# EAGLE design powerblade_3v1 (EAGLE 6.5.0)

## Sheet 1 of 6: AC-DC Power Supply
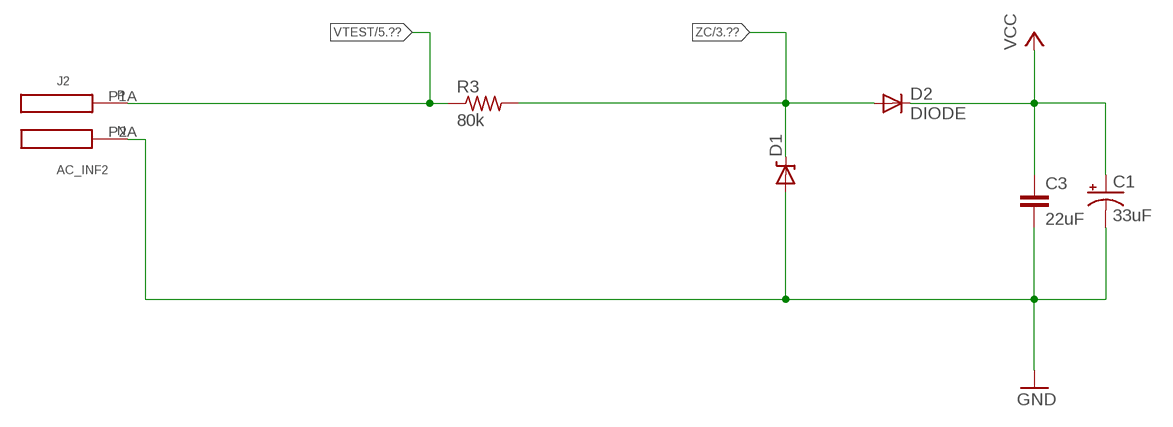
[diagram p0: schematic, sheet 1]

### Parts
C1  33uF  CPOL-US0805_SM  [CPOL0805_SM]
C3  22uF  C-EUC0603_SM  [C0603_SM]
D1  ZENERBZT52  [BZT52]
D2  DIODE  [BAS521]
J2  AC_INF2  [AC3_F2]
R3  80k  R-US_R1210  [R1210]

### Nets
GND: C1.- C3.2 D1.A J2.P2A(N) ; also sheet 2,3,4,5,6
VCC: C1.+ C3.1 D2.C ; also sheet 2,3,6
VTEST: J2.P1A(P) R3.1 ; also sheet 5
ZC: D1.C D2.A R3.2 ; also sheet 3,6

## Sheet 2 of 6: Load Supply Regulation
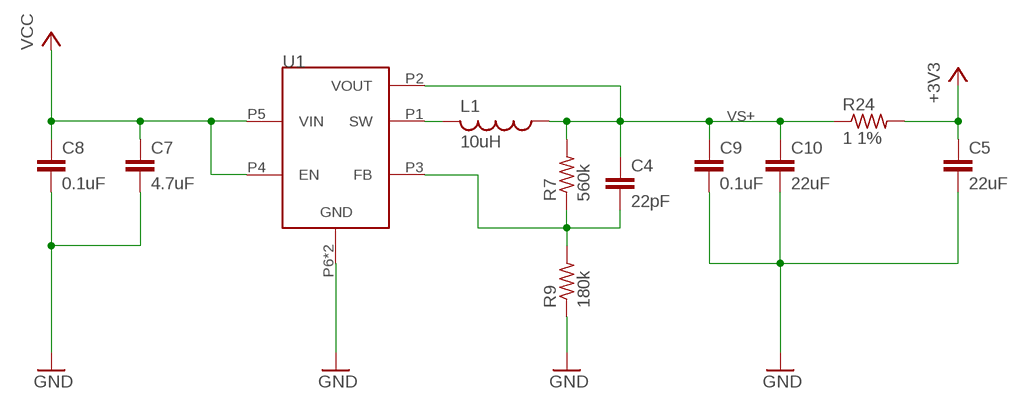
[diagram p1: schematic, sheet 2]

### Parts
C4  22pF  C-EUC0402_SM  [C0402_SM]
C5  22uF  C-EUC0603_TN  [C0603_TN]
C7  4.7uF  C-EUC0402_SM  [C0402_SM]
C8  0.1uF  C-EUC0402_SM  [C0402_SM]
C9  0.1uF  C-EUC0402_SM  [C0402_SM]
C10  22uF  C-EUC0603_SM  [C0603_SM]
L1  10uH  L-USL0805  [L0805]
R7  560k  R-US_R0402_SM  [R0402_SM]
R9  180k  R-US_R0402_SM  [R0402_SM]
R24  1 1%  R-US_R0603_SM  [R0603_SM]
U1  TPS62122  [WDFN-6]

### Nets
+3V3: C5.1 R24.2 ; also sheet 3,4,5,6
GND: C5.2 C7.2 C8.2 C9.2 C10.2 R9.1 U1.P6(GND) U1.PAD(GND) ; also sheet 1,3,4,5,6
N$9: L1.2 U1.P1(SW)
N$13: C4.2 R7.1 R9.2 U1.P3(FB)
VCC: C7.1 C8.1 U1.P4(EN) U1.P5(VIN) ; also sheet 1,3,6
VS+: C4.1 C9.1 C10.1 L1.1 R7.2 R24.1 U1.P2(VOUT) ; also sheet 6

## Sheet 3 of 6: MSP430FR5738
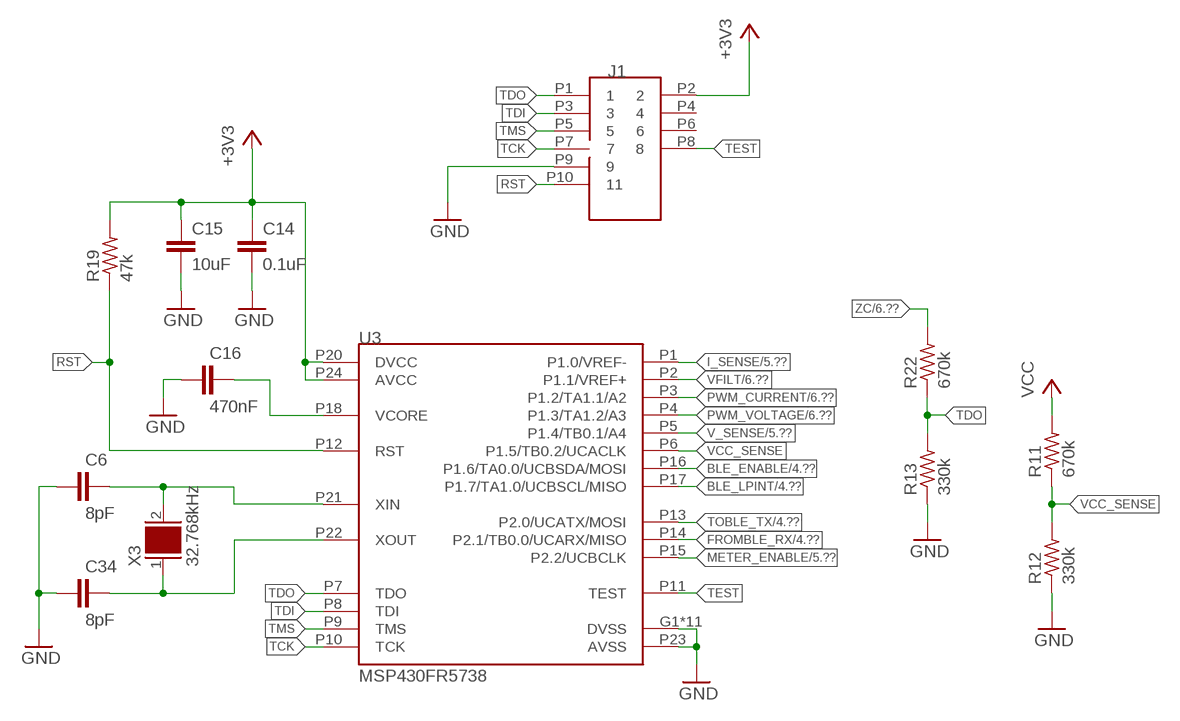
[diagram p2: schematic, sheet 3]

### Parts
C6  8pF  C-EUC0402_SM  [C0402_SM]
C14  0.1uF  C-EUC0402_SM  [C0402_SM]
C15  10uF  C-EUC0603_SM  [C0603_SM]
C16  470nF  C-EUC0402_SM  [C0402_SM]
C34  8pF  C-EUC0402_SM  [C0402_SM]
J1  JTAG_14PIN_IDC-ND  [TC2050-IDC-NL-430-ND]
R11  670k  R-US_R0402_SM  [R0402_SM]
R12  330k  R-US_R0402_SM  [R0402_SM]
R13  330k  R-US_R0402_SM  [R0402_SM]
R19  47k  R-US_R0402_SM  [R0402_SM]
R22  670k  R-US_R0402_SM  [R0402_SM]
U3  MSP430FR5738  [VQFN-24]
X3  32.768kHz  CRYSTAL_0805  [0805]

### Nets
+3V3: C14.1 C15.1 J1.P2 R19.2 U3.P20(DVCC) U3.P24(AVCC) ; also sheet 2,4,5,6
BLE_ENABLE: U3.P16(P1.6/TA0.0/UCBSDA/MOSI) ; also sheet 4
BLE_LPINT: U3.P17(P1.7/TA1.0/UCBSCL/MISO) ; also sheet 4
FROMBLE_RX: U3.P14(P2.1/TB0.0/UCARX/MISO) ; also sheet 4,6
GND: C6.1 C14.2 C15.2 C16.1 C34.1 J1.P9 R12.1 R13.1 U3.G1(DVSS) U3.G2(DVSS) U3.G3(DVSS) U3.G4(DVSS) U3.G5(DVSS) U3.G6(DVSS) U3.G7(DVSS) U3.G8(DVSS) U3.G9(DVSS) U3.P19(DVSS) U3.P23(AVSS) U3.PAD(DVSS) ; also sheet 1,2,4,5,6
I_SENSE: U3.P1(P1.0/VREF-) ; also sheet 5,6
METER_ENABLE: U3.P15(P2.2/UCBCLK) ; also sheet 5
N$3: C34.2 U3.P22(XOUT) X3.1
N$23: C16.2 U3.P18(VCORE)
N$56: C6.2 U3.P21(XIN) X3.2
PWM_CURRENT: U3.P3(P1.2/TA1.1/A2) ; also sheet 6
PWM_VOLTAGE: U3.P4(P1.3/TA1.2/A3) ; also sheet 6
RST: J1.P10 R19.1 U3.P12(RST)
TCK: J1.P7 U3.P10(TCK)
TDI: J1.P3 U3.P8(TDI)
TDO: J1.P1 R13.2 R22.1 U3.P7(TDO)
TEST: J1.P8 U3.P11(TEST)
TMS: J1.P5 U3.P9(TMS)
TOBLE_TX: U3.P13(P2.0/UCATX/MOSI) ; also sheet 4,6
V_SENSE: U3.P5(P1.4/TB0.1/A4) ; also sheet 5,6
VCC: R11.2 ; also sheet 1,2,6
VCC_SENSE: R11.1 R12.2 U3.P6(P1.5/TB0.2/UCACLK)
VFILT: U3.P2(P1.1/VREF+) ; also sheet 5,6
ZC: R22.2 ; also sheet 1,6
Unconnected: J1.P4 J1.P6

## Sheet 4 of 6: nr51822
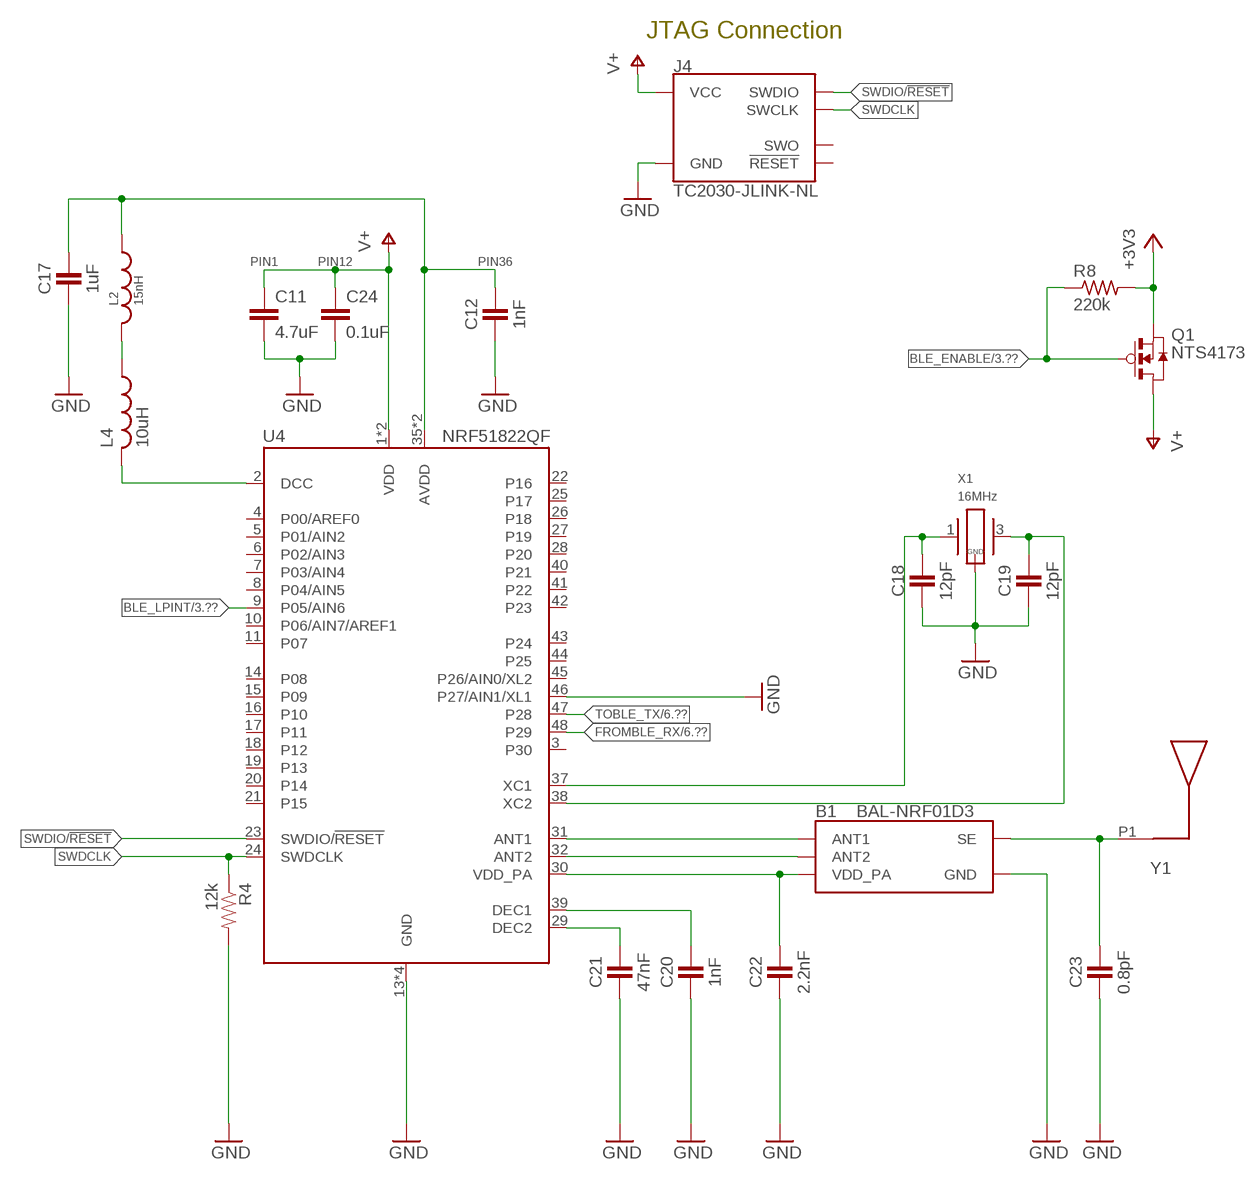
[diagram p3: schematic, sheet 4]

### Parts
B1  BAL-NRF01D3  [BAL-NRF01D3]
C11  4.7uF  C-EUC0402_SM  [C0402_SM]
C12  1nF  CAPACITOR  [0402_CAP]
C17  1uF  CAPACITOR  [0402_CAP]
C18  12pF  CAPACITOR  [0402_CAP]
C19  12pF  CAPACITOR  [0402_CAP]
C20  1nF  CAPACITOR  [0402_CAP]
C21  47nF  CAPACITOR  [0402_CAP]
C22  2.2nF  CAPACITOR  [0402_CAP]
C23  0.8pF  CAPACITOR  [0402_CAP]
C24  0.1uF  C-EUC0402_SM  [C0402_SM]
J4  TC2030-JLINK-NL  [TC2030-IDC-NL]
L2  15nH  INDUCTOR0402  [0402_CAP]
L4  10uH  L-USL0603_TN  [C0603_TN]
Q1  NTS4173  [SC-70-3]
R4  12k  RESISTOR  [0402_RES]
R8  220k  R-US_R0402_SM  [R0402_SM]
U4  NRF51822QF  [QFN-48-6MM]
X1  16MHz  TXC-8Y  [TXC-8Y]
Y1  UREACH_XTEND  [UREACH_XTEND]

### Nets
+3V3: Q1.P2(S) R8.2 ; also sheet 2,3,5,6
AVDD: C12.1 C17.1 L2.1 U4.35(AVDD) U4.36(AVDD)
BLE_ENABLE: Q1.P1(G) R8.1 ; also sheet 3
BLE_LPINT: U4.9(P05/AIN6) ; also sheet 3
DCC: L4.2 U4.2(DCC)
FROMBLE_RX: U4.48(P29) ; also sheet 3,6
GND: B1.GND C11.2 C12.2 C17.2 C18.2 C19.2 C20.2 C21.2 C22.2 C23.2 C24.2 J4.5(GND) R4.2 U4.13(GND) U4.33(GND) U4.34(GND) U4.46(P27/AIN1/XL1) U4.GND X1.2(GND) X1.4(GND) ; also sheet 1,2,3,5,6
N$4: B1.SE C23.1 Y1.P1
N$5: B1.ANT1 U4.31(ANT1)
N$6: B1.ANT2 U4.32(ANT2)
N$10: L2.2 L4.1
N$16: C18.1 U4.37(XC1) X1.1
N$17: C19.1 U4.38(XC2) X1.3
N$18: C20.1 U4.39(DEC1)
N$19: C21.1 U4.29(DEC2)
SWDCLK: J4.4(SWCLK) R4.1 U4.24(SWDCLK)
SWDIO/!RESET: J4.2(SWDIO) U4.23(SWDIO/!RESET)
TOBLE_TX: U4.47(P28) ; also sheet 3,6
V+: C11.1 C24.1 J4.1(VCC) Q1.P3(D) U4.1(VDD) U4.12(VDD)
VDD_PA: B1.VCC(VDD_PA) C22.1 U4.30(VDD_PA)
Unconnected: J4.3(!RESET) J4.6(SWO) U4.3(P30) U4.4(P00/AREF0) U4.5(P01/AIN2) U4.6(P02/AIN3) U4.7(P03/AIN4) U4.8(P04/AIN5) U4.10(P06/AIN7/AREF1) U4.11(P07) U4.14(P08) U4.15(P09) U4.16(P10) U4.17(P11) U4.18(P12) U4.19(P13) U4.20(P14) U4.21(P15) U4.22(P16) U4.25(P17) U4.26(P18) U4.27(P19) U4.28(P20) U4.40(P21) U4.41(P22) U4.42(P23) U4.43(P24) U4.44(P25) U4.45(P26/AIN0/XL2)

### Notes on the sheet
- JTAG Connection
- PIN1 | PIN12 | PIN36

## Sheet 5 of 6: Power Sensing!
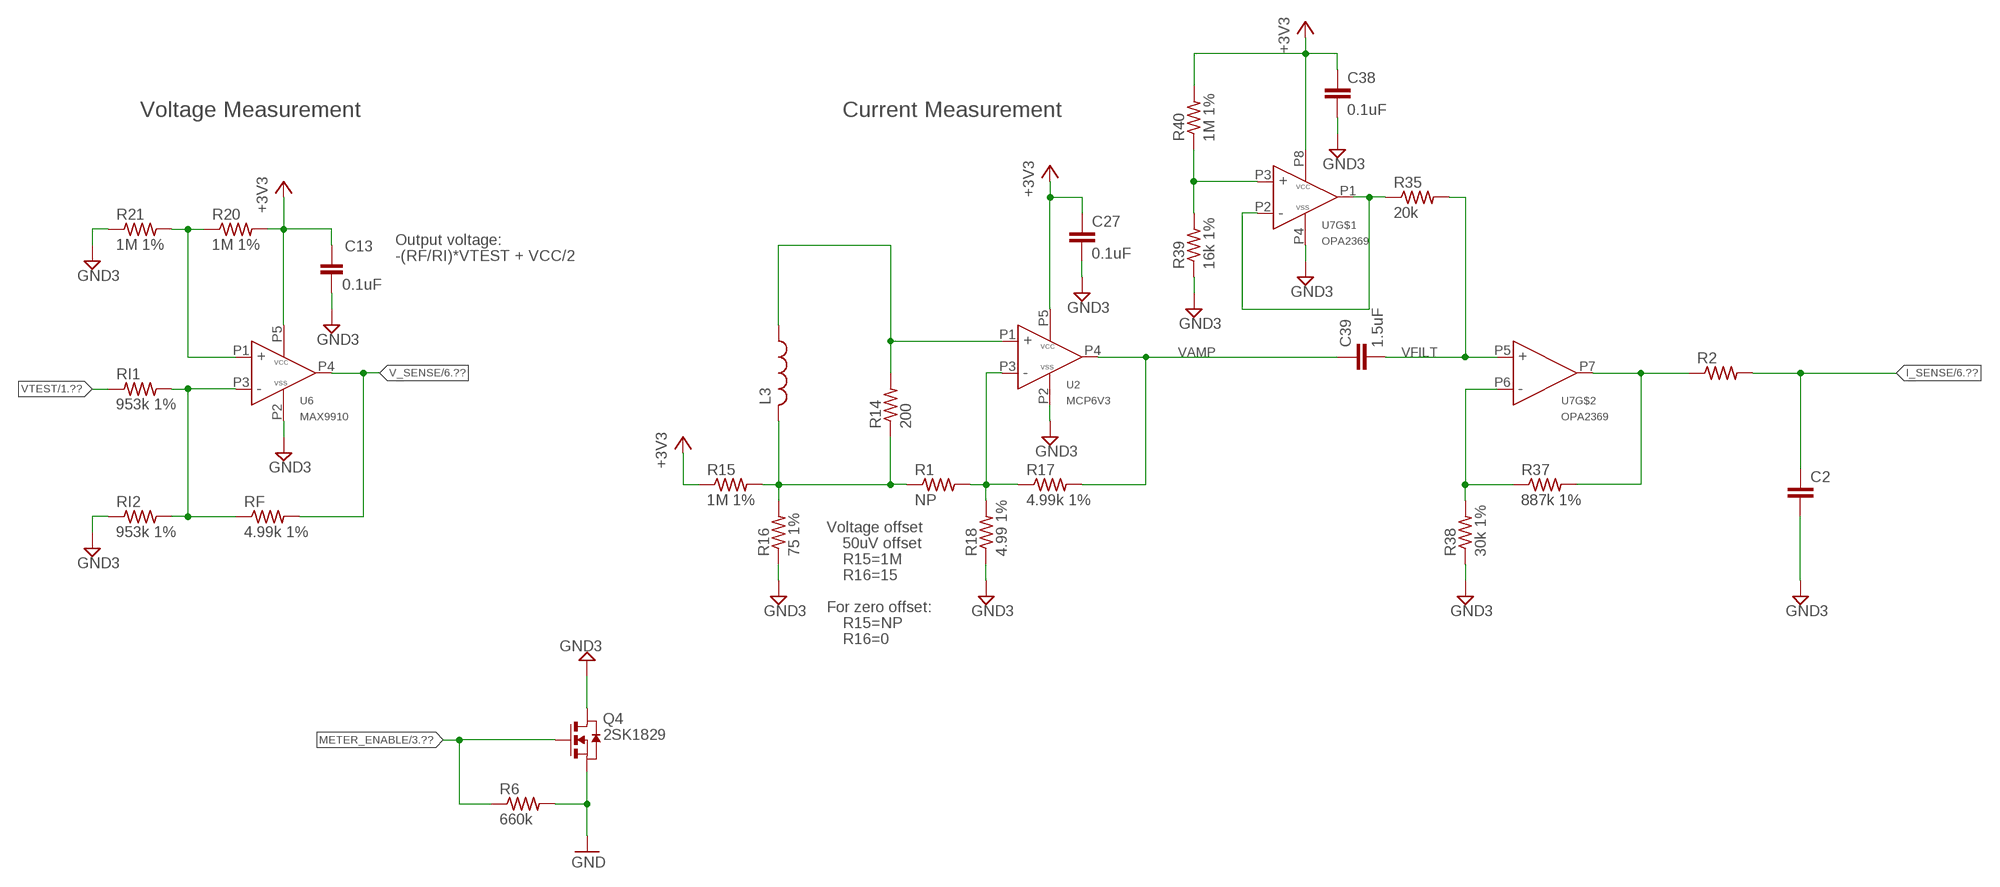
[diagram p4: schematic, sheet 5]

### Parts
C2  C-EUC0402_SM  [C0402_SM]
C13  0.1uF  CAPACITOR  [0402_CAP]
C27  0.1uF  C-EUC0402_SM  [C0402_SM]
C38  0.1uF  C-EUC0402_SM  [C0402_SM]
C39  1.5uF  C-EUC0402_SM  [C0402_SM]
L3  L-USL0805  [L0805]
Q4  2SK1829  [SC-70-3]
R1  NP  R-US_R0402_SM  [R0402_SM]
R2  R-US_R0402_SM  [R0402_SM]
R6  660k  R-US_R0402_SM  [R0402_SM]
R14  200  R-US_R0402_SM  [R0402_SM]
R15  1M 1%  R-US_R0402_SM  [R0402_SM]
R16  75 1%  R-US_R0402_SM  [R0402_SM]
R17  4.99k 1%  R-US_R0402_SM  [R0402_SM]
R18  4.99 1%  R-US_R0402_SM  [R0402_SM]
R20  1M 1%  R-US_R0402_SM  [R0402_SM]
R21  1M 1%  R-US_R0402_SM  [R0402_SM]
R35  20k  R-US_R0402_SM  [R0402_SM]
R37  887k 1%  R-US_R0402_SM  [R0402_SM]
R38  30k 1%  R-US_R0402_SM  [R0402_SM]
R39  16k 1%  R-US_R0402_SM  [R0402_SM]
R40  1M 1%  R-US_R0402_SM  [R0402_SM]
RF  4.99k 1%  R-US_R0402_SM  [R0402_SM]
RI1  953k 1%  R-US_R0402_SM  [R0402_SM]
RI2  953k 1%  R-US_R0402_SM  [R0402_SM]
U2  MCP6V3  [SC70-5]
U6  MAX9910  [SC70-5]
U7  OPA2369  [SOT-23-8]

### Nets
+3V3: C13.1 C27.1 C38.1 R15.1 R20.2 R40.2 U2.P5(VCC) U6.P5(VCC) U7.P8(VCC) ; also sheet 2,3,4,6
GND: Q4.P2(S) R6.2 ; also sheet 1,2,3,4,6
GND3: C2.2 C13.2 C27.2 C38.2 Q4.P3(D) R16.1 R18.1 R21.1 R38.1 R39.1 RI2.1 U2.P2(VSS) U6.P2(VSS) U7.P4(VSS)
I_SENSE: C2.1 R2.2 ; also sheet 3,6
METER_ENABLE: Q4.P1(G) R6.1 ; also sheet 3
N$1: R2.1 R37.2 U7.P7(OUT)
N$37: L3.2 R1.1 R14.1 R15.2 R16.2
N$38: L3.1 R14.2 U2.P1(IN+)
N$40: R20.1 R21.2 U6.P1(IN+)
N$41: RF.1 RI1.2 RI2.2 U6.P3(IN-)
N$65: R1.2 R17.1 R18.2 U2.P3(IN-)
N$66: R37.1 R38.2 U7.P6(IN-)
N$68: R35.1 U7.P1(OUT) U7.P2(IN-)
N$70: R39.2 R40.1 U7.P3(IN+)
V_SENSE: RF.2 U6.P4(OUT) ; also sheet 3,6
VAMP: C39.1 R17.2 U2.P4(OUT)
VFILT: C39.2 R35.2 U7.P5(IN+) ; also sheet 3,6
VTEST: RI1.1 ; also sheet 1

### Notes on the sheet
- Voltage Measurement | Current Measurement
- Output voltage:
- -(RF/RI)*VTEST + VCC/2
- Voltage offset
- 50uV offset
- R15=1M
- R16=15
- For zero offset:
- R15=NP
- R16=0

## Sheet 6 of 6: Debugging Connector. OOF
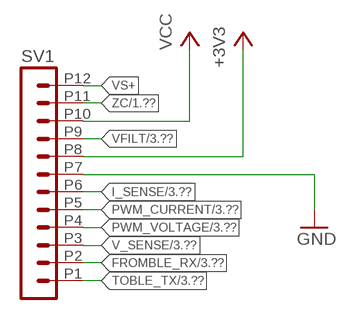
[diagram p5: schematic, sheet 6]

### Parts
SV1  MA12-11M27  [MA12-1_1MM27]

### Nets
+3V3: SV1.P8 ; also sheet 2,3,4,5
FROMBLE_RX: SV1.P2 ; also sheet 3,4
GND: SV1.P7 ; also sheet 1,2,3,4,5
I_SENSE: SV1.P6 ; also sheet 3,5
PWM_CURRENT: SV1.P5 ; also sheet 3
PWM_VOLTAGE: SV1.P4 ; also sheet 3
TOBLE_TX: SV1.P1 ; also sheet 3,4
V_SENSE: SV1.P3 ; also sheet 3,5
VCC: SV1.P10 ; also sheet 1,2,3
VFILT: SV1.P9 ; also sheet 3,5
VS+: SV1.P12 ; also sheet 2
ZC: SV1.P11 ; also sheet 1,3

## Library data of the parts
B1 = chips:BAL-NRF01D3: 50 ohm nominal input / conjugate match balun to nRF51422-QFAA, nRF24LE1, nRF51822-QFAA/AB, with integrated harmonic filter; DIGIKEY: 497-13637-1-ND; MOUSER: 511-BAL-NRF01D3
C1 = rcl:CPOL-US: POLARIZED CAPACITOR, American symbol; DIGIKEY: 478-8650-1-ND; DIGIKEY_2: 478-8654-1-ND
C2 = rcl:C-EU: CAPACITOR, European symbol
C3 C5 C10 = rcl:C-EU: CAPACITOR, European symbol; DIGIKEY: 445-9077-1-ND
C4 = rcl:C-EU: CAPACITOR, European symbol; DIGIKEY: 445-1239-1-ND
C6 C34 = rcl:C-EU: CAPACITOR, European symbol; DIGIKEY: 445-4890-1-ND
C7 = rcl:C-EU: CAPACITOR, European symbol; DIGIKEY: 445-8023-1-ND
C8 C9 C14 C24 C27 C38 = rcl:C-EU: CAPACITOR, European symbol; DIGIKEY: 445-4952-1-ND
C11 = rcl:C-EU: CAPACITOR, European symbol; DIGIKEY: 445-5947-1-ND
C12 C20 = passives:CAPACITOR: 0402 Capacitor; DIGIKEY: 490-1303-1-ND
C13 = passives:CAPACITOR: 0402 Capacitor; DIGIKEY: 445-4952-1-ND
C15 = rcl:C-EU: CAPACITOR, European symbol; DIGIKEY: 445-6853-1-ND
C16 = rcl:C-EU: CAPACITOR, European symbol; DIGIKEY: 445-4989-1-ND
C17 = passives:CAPACITOR: 0402 Capacitor; DIGIKEY: 1276-1513-1-ND
C18 C19 = passives:CAPACITOR: 0402 Capacitor; DIGIKEY: 490-6197-1-ND
C21 = passives:CAPACITOR: 0402 Capacitor; DIGIKEY: 445-1264-1-ND
C22 = passives:CAPACITOR: 0402 Capacitor; DIGIKEY: 490-5419-1-ND
C23 = passives:CAPACITOR: 0402 Capacitor; DIGIKEY: 490-6269-1-ND
C39 = rcl:C-EU: CAPACITOR, European symbol; DIGIKEY: 445-13815-1-ND
D1 = powerfilm:ZENER; DIGIKEY: BZT52C10T-7DICT-ND
D2 = powerfilm:DIODE; DIGIKEY: BAS521-7DICT-ND
J1 = ibat:JTAG_14PIN; DIGIKEY: NP
J2 = powerfilm:AC_IN; DIGIKEY: NP
J4 = connector:TC2030-JLINK; DIGIKEY: NP
L1 = rcl:L-US: INDUCTOR, American symbol; DIGIKEY: 490-4990-1-ND
L2 = passives:INDUCTOR; DIGIKEY: 587-1521-1-ND
L3 = rcl:L-US: INDUCTOR, American symbol; DIGIKEY: 732-3452-1-ND
L4 = rcl:L-US: INDUCTOR, American symbol; DIGIKEY: 490-4025-1-ND
Q1 = powerfilm:NTS4173; DIGIKEY: NTS4173PT1GOSCT-ND
Q4 = powerfilm:2SK1829; DIGIKEY: 2SK1829TE85LFCT-ND
R1 = rcl:R-US_: RESISTOR, American symbol; DIGIKEY: NP; DIGIKEY_2: P0.0JCT-ND
R2 = rcl:R-US_: RESISTOR, American symbol
R3 = rcl:R-US_: RESISTOR, American symbol; DIGIKEY: P80.6KAACT-ND; DIGIKEY_2: P69.8KAACT-ND; DIGIKEY_3: P40.2KAACT-ND
R4 = passives:RESISTOR: Resistor; DIGIKEY: RHM12.0KCDCT-ND
R6 R11 R22 = rcl:R-US_: RESISTOR, American symbol; DIGIKEY: P665KLCT-ND
R7 = rcl:R-US_: RESISTOR, American symbol; DIGIKEY: P560KLCT-ND
R8 = rcl:R-US_: RESISTOR, American symbol; DIGIKEY: P220KJCT-ND
R9 = rcl:R-US_: RESISTOR, American symbol; DIGIKEY: P180KLCT-ND
R12 R13 = rcl:R-US_: RESISTOR, American symbol; DIGIKEY: P330KLCT-ND
R14 = rcl:R-US_: RESISTOR, American symbol; DIGIKEY: P200LCT-ND
R15 R20 R21 R40 = rcl:R-US_: RESISTOR, American symbol; DIGIKEY: P1.00MLCT-ND
R16 = rcl:R-US_: RESISTOR, American symbol; DIGIKEY: P75.0LCT-ND
R17 = rcl:R-US_: RESISTOR, American symbol; DIGIKEY: P4.99KLCT-ND; DIGIKEY_2: P10.0KLCT-ND
R18 = rcl:R-US_: RESISTOR, American symbol; DIGIKEY: RMCF0402FT4R99CT-ND; DIGIKEY_2: P10.0LCT-ND
R19 = rcl:R-US_: RESISTOR, American symbol; DIGIKEY: P47KJCT-ND
R24 = rcl:R-US_: RESISTOR, American symbol; DIGIKEY: P1.0AJCT-ND
R35 = rcl:R-US_: RESISTOR, American symbol; DIGIKEY: P2.00KLCT-ND; DIGIKEY_2: P20.0KLCT-ND
R37 = rcl:R-US_: RESISTOR, American symbol; DIGIKEY: P887KLCT-ND
R38 = rcl:R-US_: RESISTOR, American symbol; DIGIKEY: P30.0KLCT-ND
R39 = rcl:R-US_: RESISTOR, American symbol; DIGIKEY: P16.0KLCT-ND
RF = rcl:R-US_: RESISTOR, American symbol; DIGIKEY: P4.99KLCT-ND
RI1 RI2 = rcl:R-US_: RESISTOR, American symbol; DIGIKEY: P953KLCT-ND
SV1 = con-lstb:MA12-1: PIN HEADER; DIGIKEY: S9014E-12-ND
U1 = powerfilm:TPS62122; DIGIKEY: 296-27695-1-ND
U2 = powerfilm:MCP6V3; DIGIKEY: MCP6V31UT-E/LTCT-ND; DIGIKEY_POP: 296-19547-1-ND
U3 = powerfilm:MSP430FR5738; DIGIKEY: 296-29232-1-ND
U4 = chips:NRF51822: Multiprotocol Bluetooth® 4.0 low energy/2.4 GHz RF SoC; DIGIKEY: 1490-1032-1-ND; MOUSER: 949-NRF51822-QFAB-R7
U6 = powerfilm:MAX9910; DIGIKEY: 296-25252-1-ND
U7 = powerfilm:OPA2369; DIGIKEY: 296-22671-1-ND
X1 = crystals:TXC-8Y: 2mmx1.6mm SMD Crystal; DIGIKEY: 887-2003-1-ND
X3 = general:CRYSTAL_0805; DIGIKEY: 535-12373-1-ND
Y1 = powerfilm:UREACH_XTEND; FRACTUS: FR05-S1-N-0-110

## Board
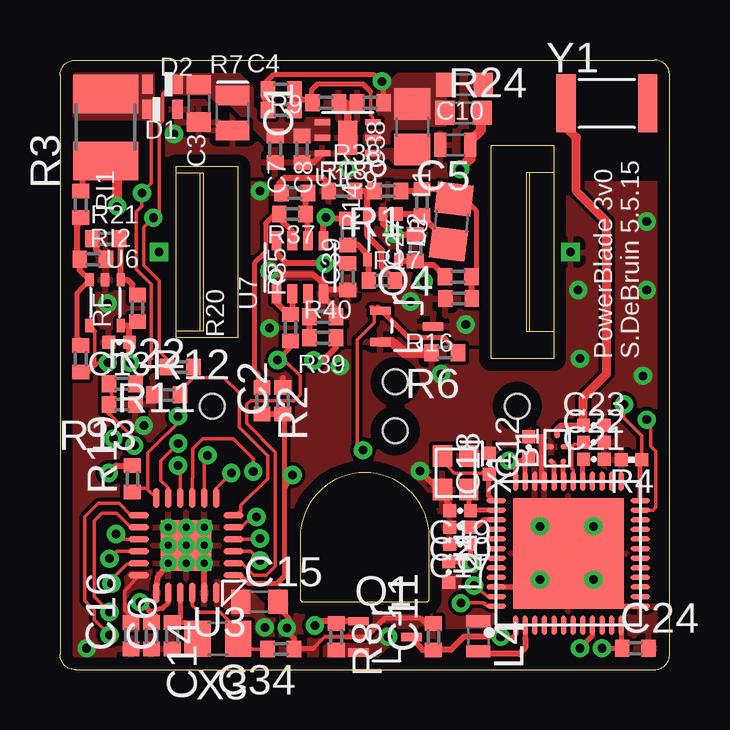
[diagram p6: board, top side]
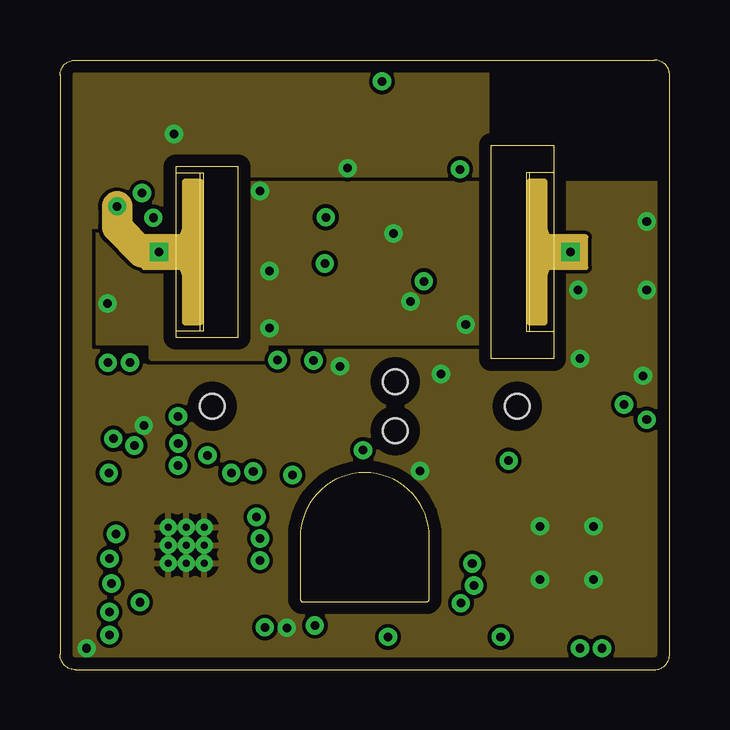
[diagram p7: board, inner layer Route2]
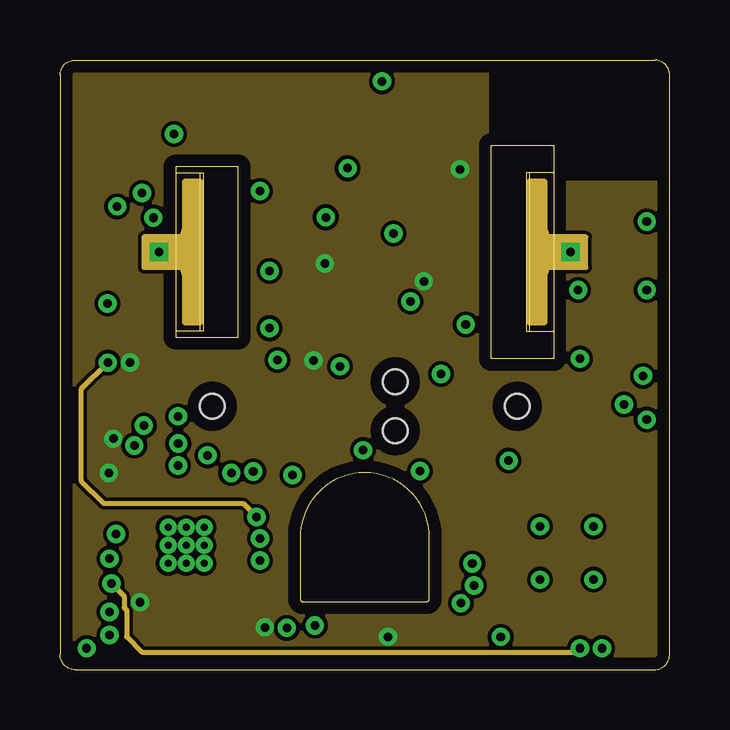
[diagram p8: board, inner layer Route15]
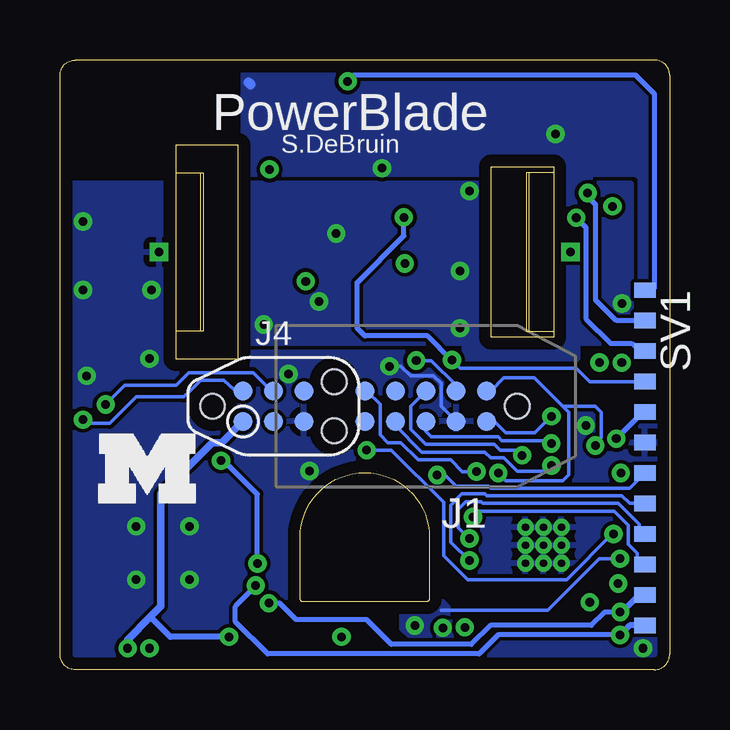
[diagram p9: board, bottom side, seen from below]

Size 25.4 x 25.4 mm. Coordinates in mm from the lower left corner, seen from the top.
Copper layers (1+2*15+16): Top 0.0178mm / dielectric 12mil / Route2 0.0356mm / dielectric 28mil / Route15 0.0356mm / dielectric 12mil / Bottom 0.0178mm
Design rules "SSC-EAGLE-4Lyr_v1.0.0.3 *": minimum track width 6mil, minimum drill 8mil, track to track 6mil, track to pad 6mil, pad to pad 6mil, via to via 6mil, smd to smd 6mil, copper to edge 20mil, drill to drill 16mil, minimum pad ring 8mil, minimum via ring 8mil, stop-mask expansion 3mil, vias tented up to drill 0mil, thermal gap 10mil

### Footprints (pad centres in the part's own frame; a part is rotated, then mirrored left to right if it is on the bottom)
BAL-NRF01D3 = smd 0.22 x 0.22: ANT1 -0.537,-0.25; ANT2 -0.537,0.25; GND 0.069,0.25; SE 0.537,0; VCC 0.069,-0.25
CPOL0805_SM = smd 0.8 x 1.4: + -0.73,0; - 0.73,0
C0402_SM = smd 0.6 x 0.7: 1 -0.55,0; 2 0.55,0
C0603_SM = smd 0.8 x 1: 1 -0.775,0; 2 0.775,0
C0603_TN = smd 0.5 x 1: 1 -0.625,0; 2 0.625,0
0402_CAP = smd 0.536 x 0.546: 1 -0.433,0; 2 0.433,0
BZT52 = smd 0.45 x 0.8: A -0.625,0; C 0.625,0
BAS521 = smd 0.45 x 0.8: A -0.625,0; C 0.625,0
TC2050-IDC-NL-430-ND = smd 0.787 x 0.787: P1 -2.54,-0.635; P2 -1.27,-0.635; P3 0,-0.635; P4 1.27,-0.635; P5 2.54,-0.635; P6 2.54,0.635; P7 1.27,0.635; P8 0,0.635; P9 -1.27,0.635; P10 -2.54,0.635 | hole 1.029: -3.81,0
AC3_F2 = drill 0.356 square: P1A -8.572,0; P2A 8.572,0
TC2030-IDC-NL = smd 0.787 x 0.787: 1 -1.27,-0.635; 2 -1.27,0.635; 3 0,-0.635; 4 0,0.635; 5 1.27,-0.635; 6 1.27,0.635 | hole 1.016: -2.54,0; 2.54,1.016; 2.54,-1.016
L0805 = smd 1.3 x 1.5: 1 -0.95,0; 2 0.95,0
SC-70-3 = smd 0.85 x 0.35: P1 -1.1,0.65; P2 -1.1,-0.65; P3 1.1,0
R0402_SM = smd 0.6 x 0.7: 1 -0.55,0; 2 0.55,0
R1210 = smd 1.6 x 2.7: 1 -1.4,0; 2 1.4,0
0402_RES = smd 0.536 x 0.546: 1 -0.433,0; 2 0.433,0
R0603_SM = smd 0.8 x 1: 1 -0.775,0; 2 0.775,0
MA12-1_1MM27 = smd 0.889 x 0.635: P1 0,6.985; P2 0,5.715; P3 0,4.445; P4 0,3.175; P5 0,1.905; P6 0,0.635; P7 0,-0.635; P8 0,-1.905; P9 0,-3.175; P10 0,-4.445; P11 0,-5.715; P12 0,-6.985
WDFN-6 = smd 0.65 x 0.25: P1 -1.05,0.65; P2 -1.05,0; P3 -1.05,-0.65; P4 1.05,-0.65; P5 1.05,0; P6 1.05,0.65 | smd 0.8 x 1.4: PAD 0,0
SC70-5 = smd 0.55 x 0.35: P1 -0.95,0.65; P2 -0.95,0; P3 -0.95,-0.65; P4 0.95,-0.65; P5 0.95,0.65
VQFN-24 = drill 0.3 pad 0.5: G1 -0.75,0.75; G2 0,0.75; G3 0.75,0.75; G4 -0.75,0; G5 0,0; G6 0.75,0; G7 -0.75,-0.75; G8 0,-0.75; G9 0.75,-0.75 | smd 0.85 x 0.28: P1 -1.975,1.25; P2 -1.975,0.75; P3 -1.975,0.25; P4 -1.975,-0.25; P5 -1.975,-0.75; P6 -1.975,-1.25; P13 1.975,-1.25; P14 1.975,-0.75; P15 1.975,-0.25; P16 1.975,0.25; P17 1.975,0.75; P18 1.975,1.25 | smd 0.28 x 0.85: P7 -1.25,-1.975; P8 -0.75,-1.975; P9 -0.25,-1.975; P10 0.25,-1.975; P11 0.75,-1.975; P12 1.25,-1.975; P19 1.25,1.975; P20 0.75,1.975; P21 0.25,1.975; P22 -0.25,1.975; P23 -0.75,1.975; P24 -1.25,1.975 | smd 2.1 x 2.1: PAD 0,0
QFN-48-6MM = smd 0.8 x 0.203: 1 -3,2.2; 2 -3,1.8; 3 -3,1.4; 4 -3,1; 5 -3,0.6; 6 -3,0.2; 7 -3,-0.2; 8 -3,-0.6; 9 -3,-1; 10 -3,-1.4; 11 -3,-1.8; 12 -3,-2.2; 25 3,-2.2; 26 3,-1.8; 27 3,-1.4; 28 3,-1; 29 3,-0.6; 30 3,-0.2; 31 3,0.2; 32 3,0.6; 33 3,1; 34 3,1.4; 35 3,1.8; 36 3,2.2 | smd 0.203 x 0.8: 13 -2.2,-3; 14 -1.8,-3; 15 -1.4,-3; 16 -1,-3; 17 -0.6,-3; 18 -0.2,-3; 19 0.2,-3; 20 0.6,-3; 21 1,-3; 22 1.4,-3; 23 1.8,-3; 24 2.2,-3; 37 2.2,3; 38 1.8,3; 39 1.4,3; 40 1,3; 41 0.6,3; 42 0.2,3; 43 -0.2,3; 44 -0.6,3; 45 -1,3; 46 -1.4,3; 47 -1.8,3; 48 -2.2,3 | smd 4.6 x 4.6: GND 0,0
SOT-23-8 = smd 0.8 x 0.4: P1 -1.1,0.975; P2 -1.1,0.325; P3 -1.1,-0.325; P4 -1.1,-0.975; P5 1.1,-0.975; P6 1.1,-0.325; P7 1.1,0.325; P8 1.1,0.975
TXC-8Y = smd 0.9 x 0.8: 1 -0.7,-0.55; 2 0.7,-0.55; 3 0.7,0.55; 4 -0.7,0.55
0805 = smd 1.1 x 1.5: 1 -0.85,0; 2 0.85,0
UREACH_XTEND = smd 0.8 x 2.4: NC 1.7,0; P1 -1.7,0

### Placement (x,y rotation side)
B1  20.72,9.22 90 top
C1  7.19,23.19 270 top
C2  9.29,11.21 90 top
C3  5.78,23.59 270 top
C4  9.22,23.32 0 top
C5  16.48,21.86 180 top
C6  4.67,1.41 90 top
C7  8.97,21.69 270 top
C8  10.08,21.69 270 top
C9  12.93,23.62 180 top
C10  16.86,24.37 0 top
C11  15.56,1.37 90 top
C12  19.53,9.27 90 top
C13  2.46,13.64 180 top
C14  3.81,1.41 270 top
C15  8.31,2.82 0 top
C16  2.96,1.42 90 top
C17  16.67,5.23 180 top
C18  17.88,8.58 90 top
C19  16.67,6.62 180 top
C20  16.67,5.92 180 top
C21  22.24,8.76 0 top
C22  22.24,9.47 0 top
C23  22.24,10.18 0 top
C24  23.98,0.89 0 top
C27  14.81,17.58 90 top
C34  9.2,0.86 180 top
C38  11.99,16.37 270 top
C39  11.99,18.24 90 top
D1  4.27,23.35 180 top
D2  4.27,24.38 0 top
J1  10.16,10.97 180 bottom
J2  12.7,17.4 0 top
J4  16.51,10.97 0 bottom
L1  14.68,22.62 270 top
L2  16.19,4.06 270 top
L3  16.31,18.67 82.9 top
L4  17.43,1.4 270 top
Q1  13.54,1.37 0 top
Q4  14.45,14.3 0 top
R1  13.65,19.94 180 top
R2  8.41,11.21 270 top
R3  1.9,22.59 90 top
R4  23.81,8.75 180 top
R6  16.03,13.21 180 top
R7  9.22,24.17 180 top
R8  11.51,1.37 270 top
R9  11.07,23.62 180 top
R11  5.02,12.61 180 top
R12  4.44,11.45 0 top
R13  2.59,11.05 180 top
R14  15.08,19.46 270 top
R15  16.59,16.37 0 top
R16  16.61,15.46 0 top
R17  13.41,16.21 180 top
R18  11.75,19.94 0 top
R19  3.02,7.95 90 top
R20  3.23,15.06 270 top
R21  1.9,17.95 0 top
R22  2.59,11.91 0 top
R24  16.81,23.19 0 top
R35  9.6,14.25 270 top
R37  9.68,18.99 180 top
R38  9.78,19.86 0 top
R39  10.95,14.7 180 top
R40  10.95,13.83 0 top
RF  0.86,12.95 270 top
RI1  0.86,19.38 270 top
RI2  1.37,17.1 180 top
SV1  1.03,8.83 180 bottom
U1  11.99,22.16 180 top
U2  13.46,18.03 270 top
U3  5.25,5.18 180 top
U4  21.18,4.84 90 top
U6  1.88,15.29 270 top
U7  10,16.76 90 top
U$1  [BLOCK-M]  23.81,6.92 0 bottom
X1  16.48,8.2 270 top
X3  6.58,1.28 180 top
Y1  22.78,23.6 0 top

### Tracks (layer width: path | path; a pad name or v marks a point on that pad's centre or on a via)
+3V3  (via drill 0.36)
  Top 0.203: U3.P20 4.5,2.77 4.29,2.56 3.97,2.48 3.85,2.36
  Top 0.254: R15.1 15.56,16.84 15.16,16.84 | U2.P5 14.17,17.03 C27.1 14.81,16.96 14.92,16.84 15.16,16.84 | v15.16,16.18 15.24,16.26 15.24,16.76 15.16,16.84 | C38.1 v11.03,16.92 9.45,16.92 9.05,17.32 9.05,17.84 U7.P8 | C14.1 3.97,2.24 3.85,2.36 3.48,2.73 v3.33,2.81 | R40.2 11.51,13.43 10.95,12.88 v10.56,12.88 | v2.92,12.8 2.89,13.06 C13.1 2.89,14.31 2.86,14.34 | U6.P5 2.86,14.34 | 2.86,14.34 2.97,14.34 3.17,14.54 3.2,14.54 R20.2 | v2.03,8.19 2.34,8.5 R19.2
  Top 0.406: v16.67,20.85 17.1,21.28 C5.1 17.1,22.04 17.54,22.48 17.54,23.15 R24.2
  Bottom 0.152: J1.P2 8.89,11.84 9.92,12.88 v10.56,12.88
  Bottom 0.203: SV1.P8 1.11,10.73 v2.22,9.62
  other vias: 8.53,1.76 13.67,1.37
  pour Route15: -0.32,-0.38 24.89,-0.38 24.89,20.26 17.78,20.26 17.78,26.29 -0.32,26.29
  pour Top (no thermals): 6.51,2.32 7.54,2.32 8.49,1.37 8.97,1.37 9.13,1.52 9.13,1.92 7.54,3.67 6.51,3.67
  pour Top (no thermals): 11.03,0.57 13.18,0.57 13.65,1.05 13.65,1.6 13.41,1.84 12.46,1.84 11.67,1.05 11.03,1.05
AVDD  (via drill 0.36)
  Top 0.203: U4.35 19.38,8.7 19.44,8.75 | 19.44,8.75 C12.1 | 19.44,8.75 19.37,8.83 19.25,8.71 19.05,8.71 | L2.1 17.1,4.5 v17.18,4.42 17.1,4.5 C17.1 | 19.05,8.71 v18.69,8.71 | U4.36 18.98,8.64 19.05,8.71
  Bottom 0.203: v17.18,4.42 17.18,7.31 18.57,8.71 v18.69,8.71
BLE_ENABLE  (via drill 0.36)
  Top 0.152: U3.P16 2.37,4.93 v2.06,4.62
  Top 0.254: Q1.P1 11.45,2.02 | 11.45,2.02 R8.1 | 11.45,2.02 10.79,2.02 v10.62,1.84
  Bottom 0.152: 9.52,2.48 5.08,2.48 2.94,4.62 v2.06,4.62
  pour Bottom (no thermals): 9.21,2.64 9.21,1.6 9.45,1.37 10.87,1.37 11.19,1.68 11.19,2.71 10.79,3.11 9.68,3.11
BLE_LPINT  (via drill 0.36)
  Top 0.152: U3.P17 2.98,4.43 2.94,4.38 2.78,4.38 2.14,3.75 v2.14,3.59
  Top 0.203: U4.9 22.18,1.4 v21.67,0.89
  Route15 0.203: v2.14,3.59 2.67,3.06 2.67,2.58 2.78,2.48 2.78,1.37 3.41,0.73 21.51,0.73 v21.67,0.89
DCC
  Top 0.203: U4.2 19.38,1.3
  Top 0.254: 19.38,1.3 19.38,0.91 19.13,0.65 17.74,0.65 L4.2
FROMBLE_RX  (via drill 0.36)
  Top 0.152: U4.48 17.85,2.64 17.62,2.79 16.73,2.79 v16.7,2.77 | v2.06,2.4 1.43,3.03 1.43,6.21 1.75,6.53 2.36,6.53 2.96,5.93 U3.P14
  Bottom 0.203: v2.06,2.4 2.7,2.4 3.25,1.84 7.46,1.84 8.25,1.05 11.59,1.05 12.62,2.08 15.56,2.08 16.25,2.77 v16.7,2.77
  Bottom 0.254: SV1.P2 1.27,3.11 1.9,2.48 1.98,2.48 v2.06,2.4
GND  (via drill 0.36)
  Top 0.152: 10.56,0.89 11.03,1.37 11.91,1.37
  Top 0.203: C15.2 9.08,2.6 9.52,2.16 9.52,1.52 9.76,1.29 9.76,0.81 9.84,0.89 10.56,0.89 | C19.2 16.24,6.88 16.11,7 16.11,7.32 X1.2 | U4.13 21.18,2.64 21.18,4.06 | 21.18,4.06 U4.GND | U4.33 20.08,7.84 20.08,9.22 20.15,9.29 B1.GND 20.46,9.3 20.08,9.3 20.08,9.7 C12.2 | U4.46 20.56,3.44 21.07,3.95 21.18,4.06 | 11.91,1.37 12.75,1.37 13.55,2.16 15,2.16 15.24,1.92 C11.2 15.54,1.92
  Top 0.254: U3.P19 4.07,3.85 U3.G3 | U1.P6 10.56,21.14 C8.2 | U3.P23 U3.G1 | X1.2 15.77,7.5 v15,8.27 | v20,3.75 20.87,3.75 21.07,3.95
  Top 0.305: U1.PAD 11.99,23.51 11.75,23.75 R9.1
  Top 0.406: Q4.P2 13.83,13.65 14.37,13.19 R6.2
  Bottom 0.152: J1.P9 9.52,10.97 9.52,11.92 9.84,12.24 10.79,12.24 11.19,12.64 v11.67,12.64
  Bottom 0.406: 17.54,24.46 17.46,24.38
  other vias: 9.45,1.74 4.75,22.32 21.67,12.95 15.88,12.32 3.49,10.17 1.11,0.89 21.59,15.81 11.99,20.89 24.29,12.24 22.23,3.75 20,5.97 22.23,5.97 24.45,18.67 24.45,15.81
  pour Top (rank 6): -1.27,26.54 17.78,26.54 17.78,20.26 24.89,20.27 24.89,-0.38 -1.27,-0.38
  pour Bottom (rank 6): -1.27,26.54 17.78,26.54 17.78,20.26 24.89,20.27 24.89,-0.38 -1.27,-0.38
  pour Route2 (rank 6): -1.27,26.54 4.13,26.54 4.13,26.53 17.78,26.54 17.78,20.26 24.89,20.27 24.89,-0.38 -1.27,-0.38
  pour Route2 (no thermals): 21.11,18.91 21.11,16.05 22.7,16.05 22.7,16.13 22.7,18.91
GND3  (via drill 0.36)
  Top 0.254: C27.2 13.94,18.13 v13.89,18.17 13.46,18.6 U2.P2 | R38.1 9.13,20.26 9.37,20.5 10.95,20.5 11.19,20.26 R18.1 | U7.P4 10.98,15.55 11.51,15.02 R39.1 | C38.2 11.13,15.82 U7.P4 | C2.2 9.29,12.16 | U7.P4 10.98,16.11 10.56,16.45 8.89,16.45 v8.73,16.61 | RI2.1 1.51,17.51 1.51,17.8 R21.1
  other vias: 14.6,15.34 16.91,14.38 8.33,19.94 8.73,14.22 1.98,15.26
  pour Bottom (rank 4): 18.1,13.59 8.57,13.59 8.57,12.95 3.81,12.95 3.81,13.59 1.59,13.59 1.59,20.26 18.1,20.26
  pour Route2 (rank 4): 18.1,13.59 8.57,13.59 8.57,12.95 3.81,12.95 3.81,13.59 1.59,13.59 1.59,20.26 18.1,20.26
  pour Top (rank 4): 18.1,13.59 8.57,13.59 8.57,12.95 3.81,12.95 3.81,13.59 1.59,13.59 1.59,20.26 18.1,20.26
  pour Top (no thermals): 9.05,11.6 9.6,11.6 9.6,12.16 9.13,12.64 9.13,13.99 9.13,14.38 8.89,14.62 8.65,14.62 8.33,14.3 8.33,12.4 9.05,11.68
I_SENSE  (via drill 0.36)
  Top 0.203: U3.P1 7.52,3.93 7.86,3.59 9.05,3.59 9.37,3.91 9.37,7.56 | 9.37,7.56 9.37,10.57 9.21,10.73 | v9.68,8.11 9.37,7.56
  Top 0.254: R2.2 9.12,10.66 9.21,10.73 9.21,10.74 C2.1
  Bottom 0.152: SV1.P6 1.67,7.56 7.46,7.56 7.54,7.64 8.89,7.64 9.37,8.11 v9.68,8.11
METER_ENABLE  (via drill 0.36)
  Top 0.152: U3.P15 2.61,5.43 v2.34,5.65 | v12.62,9.14 12.38,9.38 12.38,13.75 13.1,14.46 13.1,15.03 13.02,15.11 | 12.95,15.11 13.02,15.11 | 13.02,15.11 Q4.P1
  Top 0.203: R6.1 16.03,13.83 14.53,13.83 13.26,15.1 13.2,15.1 Q4.P1
  Bottom 0.152: v2.34,5.65 2.38,5.65 4.29,3.75 8.41,3.75 9.42,4.75 9.42,6.98 11.59,9.14 v12.62,9.14
N$1
  Top 0.203: R37.2 8.97,18.99 8.57,18.59 8.57,17.4 8.1,16.92 8.1,12.48 8.25,12.32 8.25,12 8.33,12 R2.1 8.25,12.08
  Top 0.254: U7.P7 9.68,18.28 9.21,18.75 9.21,18.91 R37.2
N$3
  Top 0.152: C34.2 8.02,0.86 X3.1 7.3,1.58 7.3,1.76 6.67,2.4 5.79,2.4 5.5,2.69 U3.P22
N$4
  Top 0.254: B1.SE 20.72,10.02 20.88,10.18 C23.1
  Top 0.381: C23.1 21.81,11.27 21.81,11.35 22.78,12.32 22.78,18.67 21.51,19.94 21.51,22.16 21.11,22.56 21.11,23.66
  Top 0.508: 21.11,23.66 Y1.P1
N$5
  Top 0.203: U4.31 20.97,7.86 B1.ANT1
N$6
  Top 0.203: U4.32 20.58,8.57 B1.ANT2
N$9
  pour Top (rank 3, no thermals): 12.7,21.37 13.73,21.37 13.97,21.13 15.32,21.13 15.32,22.24 14.21,22.24 13.57,21.61 12.7,21.61
N$10
  pour Top (rank 2, no thermals): 15.8,1.76 17.86,1.76 18.1,2 18.1,2.95 16.67,3.11 16.67,3.91 15.72,3.91 15.64,3.83 15.64,1.92
N$13
  Top 0.152: U1.P3 13.04,23.02 12.94,23.11 12.94,24.08
  Top 0.203: 12.94,24.08 12.62,24.41 10.74,24.41 10.48,24.15 10.48,23.75
  Top 0.254: R7.1 9.68,23.75 | 9.68,23.75 C4.2 | 9.68,23.75 10.48,23.75 R9.2
N$16
  Top 0.152: 17.62,8.19 16.43,8.19 16.19,8.43 16.19,8.64 X1.1
  Top 0.203: U4.37 18.06,7.04 17.86,7.24 17.86,8.12 C18.1 17.67,8.15 17.62,8.19
N$17
  Top 0.203: U4.38 17.12,6.64 | 17.12,6.64 C19.1 | X1.3 17.04,6.73 17.12,6.64
N$18
  Top 0.203: U4.39 17.66,6.24 17.38,5.97 17.15,5.97 C20.1
N$19
  Top 0.203: U4.29 21.78,8.73 C21.1
N$23
  Top 0.152: U3.P18 2.7,3.27 2.7,2.48 3.09,2.09 C16.2
  pour Top (rank 2, no thermals): 3.81,4.06 3.02,4.06 2.7,3.75 2.7,1.68 3.49,1.68 3.49,2.32 3.81,2.64
N$37
  Top 0.203: R15.2 17.36,16.59 17.36,19.09 16.83,19.62 16.51,19.62 16.5,19.61 L3.2
  Top 0.254: L3.2 16.02,20.01 R14.1 15.01,19.94 R1.1 | R15.2 17.14,15.5 17.14,15.49 17.14,15.47 R16.2
N$38
  Top 0.254: L3.1 16.19,17.8 R14.2 15.01,18.98 U2.P1
N$40
  Top 0.254: R21.2 2.46,17.8 2.54,17.72 2.54,16.25 U6.P1 2.54,16.21 2.85,16.21 3.02,16.05 3.02,15.82 R20.1
N$41
  Top 0.203: RF.1 0.86,13.68 0.71,13.83 0.71,15.69 U6.P3
  Top 0.254: U6.P3 0.82,16.65 RI2.2 0.71,17.21 0.71,18.51 0.86,18.66 RI1.2
N$56
  Top 0.203: 4.84,2.08 4.84,1.98 C6.2 | C6.2 5.22,1.96 X3.2 | U3.P21 5,2.14 C6.2
N$65
  Top 0.254: R1.2 12.7,19.94 | 12.7,19.94 R18.2 | 12.7,19.94 12.81,19.83 U2.P3 12.81,18.08 13.41,17.48 13.41,16.76 R17.1
N$66
  Top 0.254: U7.P6 10.33,18.89 R37.1 10.23,19.76 R38.2
N$68
  Top 0.254: R35.1 9.49,14.82 | 9.49,14.82 9.03,15.28 U7.P1 | U7.P2 9.68,15.01 9.49,14.82
N$70
  Top 0.254: U7.P3 10.33,14.78 R39.2 10.48,14.77 | R40.1 10.4,14.47 10.48,14.54 10.48,14.77 | 10.48,14.86 10.48,14.77
PWM_CURRENT  (via drill 0.36)
  Top 0.152: U3.P3 7.95,4.93 v8.33,4.54
  Bottom 0.152: SV1.P5 1.67,6.92 1.98,7.24 7.62,7.24 7.7,7.32 8.65,7.32 9.11,6.86 9.11,5.31 v8.33,4.54
PWM_VOLTAGE  (via drill 0.36)
  Top 0.152: U3.P4 8.3,5.43 v8.33,5.46
  Bottom 0.152: SV1.P4 1.27,5.65 1.27,6.05 2.14,6.92 7.78,6.92 7.86,7 8.49,7 8.81,6.69 8.81,5.91 v8.33,5.46
RST  (via drill 0.36)
  Top 0.152: v4.92,10.55 4.92,10.29 3.97,9.35 3.65,9.03 3.65,7.56 | 3.65,7.56 3.65,7.55 3.64,7.56 3.17,7.56 R19.1 | U3.P12 3.65,7.5 3.65,7.56
  Bottom 0.152: J1.P10 7.31,10.34 6.83,9.86 5.62,9.86 v4.92,10.55
SWDCLK  (via drill 0.36)
  Top 0.152: R4.1 24.25,9.74 23.49,10.49 v23.49,11.05
  Top 0.203: U4.24 24.18,8.69 R4.1
  Bottom 0.152: J4.4 16.64,11.65 17.36,12.37 20.03,12.37 20.56,11.84 22.7,11.84 v23.49,11.05
SWDIO/!RESET  (via drill 0.36)
  Top 0.152: U4.23 24.72,6.64 24.82,6.76 24.82,9.09 24.61,9.3 24.61,10.26 v24.45,10.41
  Bottom 0.152: J4.2 18.14,11.65 18.57,12.07 19.53,12.07 20,11.61 20.24,11.37 22.23,11.37 23.34,10.26 24.29,10.26 v24.45,10.41
TCK  (via drill 0.36)
  Top 0.152: U3.P10 5,8.35 4.96,8.4 v4.91,8.51
  Bottom 0.152: J1.P7 11.43,10.18 10.32,9.07 7.7,9.07 7.46,8.83 6.91,8.83 6.35,8.27 5.2,8.27 v4.91,8.51
TDI  (via drill 0.36)
  Top 0.152: U3.P8 6,8.79 v6.14,8.93
  Bottom 0.152: J1.P3 10.79,10.97 10.79,10.02 10.16,9.38 7.3,9.38 7.06,9.14 6.36,9.14 v6.14,8.93
TDO  (via drill 0.36)
  Top 0.152: U3.P7 6.5,7.55 v7.14,8.19 | 2.04,10.68 3.17,9.54 3.17,9.41 v3.1,9.33 | R22.1 2.23,11.24 R13.2
  Top 0.203: R13.2 2.04,10.68
  Bottom 0.152: J1.P1 7.46,11.61 6.91,12.16 5.64,12.16 4.44,10.97 | 4.44,10.97 4.21,10.73 4.21,8.11 4.44,7.87 6.83,7.87 v7.14,8.19 | v3.1,9.33 3.14,9.38 2.86,9.67 2.86,10.73 3.1,10.97 4.44,10.97
TEST  (via drill 0.36)
  Top 0.152: U3.P11 4.5,7.58 4.21,7.87 4.21,8.7 v4.93,9.42
  Bottom 0.152: J1.P8 10.16,9.94 9.92,9.7 7.14,9.7 6.98,9.54 5.05,9.54 v4.93,9.42
TMS  (via drill 0.36)
  Top 0.152: U3.P9 5.5,7.98 5.53,8.01 5.53,9.2 5.95,9.62 7.22,9.62 8.05,8.79 v8.05,8.25
  Bottom 0.152: J1.P5 12.62,11.61 12.06,11.05 12.06,9.78 11.75,9.46 11.19,9.46 10.48,8.75 9.13,8.75 8.63,8.25 v8.05,8.25
TOBLE_TX  (via drill 0.36)
  Top 0.152: v2.06,1.45 1.43,2.08 1.43,2.48 1.03,2.87 1.03,6.37 1.59,6.92 2.46,6.92 2.96,6.43 U3.P13 | U4.47 17.85,3.04 17.22,3.51
  Top 0.203: U3.P13 3.41,6.44 | 17.22,3.51 v17.25,3.51
  Bottom 0.203: v2.06,1.45 7.14,1.45 7.94,0.65 16.75,0.65 18.1,2 18.1,2.64 17.25,3.49 v17.25,3.51
  Bottom 0.254: SV1.P1 1.67,1.84 v2.06,1.45
V+  (via drill 0.36)
  Top 0.203: U4.12 23.38,0.98 C24.1 v22.58,0.89 | U4.1 18.98,1.46 18.81,1.29 18.44,1.29 v18.36,1.37
  Top 0.254: v18.36,1.37 16.83,1.37 16.28,0.82 C11.1 15.11,0.82 Q1.P3
  Bottom 0.254: v18.36,1.37 20.8,1.37 21.63,2.2
  Bottom 0.305: J4.1 18.66,9.46 19.05,9.46 21.19,7.32 21.19,2.64 21.63,2.2 22.58,1.25 v22.58,0.89
V_SENSE  (via drill 0.36)
  Top 0.152: U3.P5 7.55,5.93 8.15,6.53 v8.19,6.36 | 1.2,12.4 1.45,12.64 | 1.45,12.64 1.45,14.11 | v1.99,12.79 1.6,12.79 1.45,12.64
  Top 0.203: RF.2 1.2,12.4 | 1.45,14.11 U6.P4
  Route15 0.203: v1.99,12.79 0.87,11.68 0.87,7.87 1.83,6.92 7.63,6.92 v8.19,6.36
  Bottom 0.152: 1.27,4.38 1.35,4.46 1.35,4.86 1.72,5.23 1.72,6.02 2.3,6.6 7.95,6.6 v8.19,6.36
  Bottom 0.203: SV1.P3 1.27,4.38
VAMP
  Top 0.254: C39.1 12.02,17.72 12.38,17.72 12.81,17.29 U2.P4 12.86,17.03 R17.2
VCC  (via drill 0.36)
  Top 0.152: D2.C 4.68,24.38 4.29,23.99 4.29,22.88 4.13,22.72 4.13,18.99 4.05,18.99 v3.89,18.83 3.49,18.43 3.49,16.84 4.13,16.21 4.13,13.27 4.44,12.95 4.44,12.64 R11.2
  Bottom 0.203: SV1.P10 1.27,13.27 1.59,13.59 2.46,13.59 3.49,14.62 3.49,18.43 v3.89,18.83
  pour Top (no thermals): 11.19,22.08 10.48,22.08 10.4,22 8.65,22 7.06,23.59 6.59,23.59 6.19,23.99 4.68,23.99 4.68,24.78 7.46,24.78 8.02,24.23 8.02,23.43 8.49,22.96 11.19,22.96
VCC_SENSE
  Top 0.152: U3.P6 7.54,6.59 7.54,6.84 8.66,7.95 8.66,8.91 7.46,10.1 7.46,11.53 6.83,12.16 5.56,12.16 | R12.2 4.99,11.6 5.56,12.16 | 5.56,12.16 5.56,12.63 R11.1
VDD_PA
  Top 0.152: U4.30 21.38,8.32 21.31,8.39 21.31,9.27 21.43,9.38 21.73,9.38 C22.1
  Top 0.203: B1.VCC 21.29,9.29 21.31,9.27
VFILT  (via drill 0.36)
  Top 0.152: U3.P2 7.58,4.43 8.07,3.93 8.6,3.93 8.97,4.3 8.97,9.07 7.78,10.26 7.78,11.05 7.94,11.21 9.76,11.21 10,11.45 10,12.24 9.37,12.88 9.09,12.88 v9.07,12.9
  Top 0.203: R35.2 9.6,13.43 v9.07,12.9
  Top 0.254: U7.P5 10.98,18.75 v11.07,18.85 11.13,18.79 C39.2
  Bottom 0.152: v9.07,12.9 8.73,12.56 3.89,12.56 3.33,12 SV1.P9
  Bottom 0.203: v9.07,12.9 10.08,13.91 12.7,13.91 13.02,14.22 13.02,16.13 11.07,18.07 v11.07,18.85
VS+  (via drill 0.36)
  Top 0.203: C9.1 13.49,24.39 13.41,24.46 | 13.41,24.46 13.1,24.78 8.89,24.78 8.49,24.38 8.49,24.07 | 13.41,24.46 v13.41,24.51
  Top 0.254: C4.1 8.57,23.2 8.57,23.75 8.49,23.83 8.49,24.07 R7.2
  Bottom 0.203: v13.41,24.51 13.14,24.78 1.43,24.78 0.63,23.99 0.63,15.89 1.03,15.73 SV1.P12
  pour Top (rank 2, no thermals): 12.7,22 14.6,22 15.32,22.72 16.03,22.72 16.03,24.78 14.13,24.78 13.26,23.91 13.26,22.8 12.7,22.24
VTEST  (via drill 0.36)
  Top 0.254: RI1.1 0.95,20.02 0.95,20.89 1.25,21.19 R3.1
  Top 0.406: R3.1 2.38,20.71 v2.38,19.3
  Route2 1.27: v2.38,19.3 2.38,18.43 3.41,17.4 J2.P1A
ZC  (via drill 0.36)
  Top 0.152: D1.C 3.81,23.18 3.81,20.26 v3.41,19.86 3.41,19.3 3.18,19.07 3.18,16.68 3.81,16.05 3.81,12.95 3.73,12.88 3.73,12.56 3.17,12 3.17,11.87 | 3.33,12.08 3.33,12.01 R22.2 3.17,11.87 | 3.17,11.68 3.17,11.87
  Bottom 0.203: v3.41,19.86 3.41,19.7 3.1,19.38 3.1,15.42 2.22,14.54 SV1.P11
  pour Top (no thermals): 3.89,22.96 0.71,22.96 0.56,23.11 0.56,24.86 3.89,24.86

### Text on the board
tPlace: PowerBlade 3v0 | S.DeBruin 5.5.15
bPlace: PowerBlade | S.DeBruin

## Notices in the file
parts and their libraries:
SparkFun-Aesthetics: Licensing: CC v3.0 Share-Alike You are welcome to use this library for commercial purposes.
